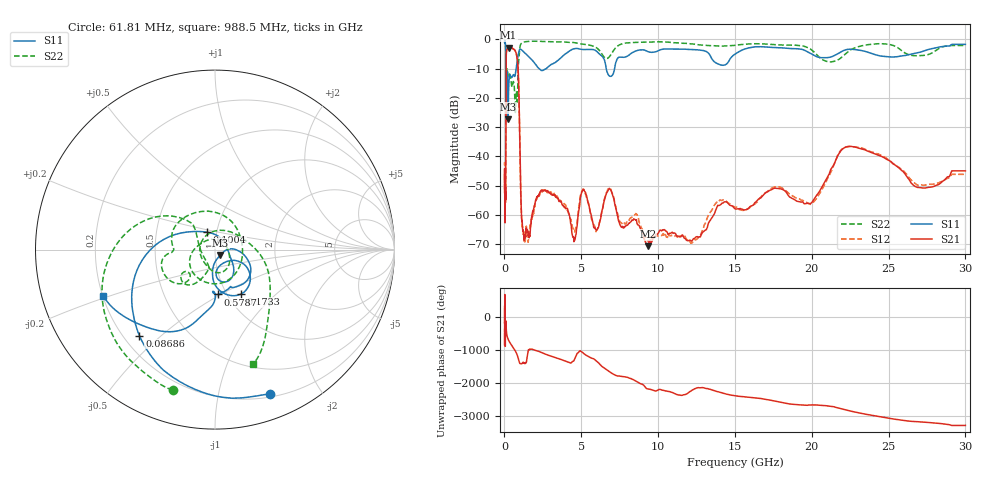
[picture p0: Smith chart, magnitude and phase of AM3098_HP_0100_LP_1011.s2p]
! Date/Time: Thu, Feb 28, 2019 8:35 AM
! Network Analyzer: Agilent Technologies E8364B Rev: A.07.50.67
! Sweep from 0.010 to 30.000 GHz, 1601 Points, Sweep Type: LOG
! Power Supply: 5.022 V, 0.002 A
# Hz S DB R 50
!freq MagS11 AngS11 MagS21 AngS21 MagS12 AngS12 MagS22 AngS22
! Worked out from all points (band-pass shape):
!   1601 points, 10 MHz to 30 GHz, reference 50 ohm
!   highest |S21| = -2.82 dB at 270.5 MHz (marker M1); lowest = -70.7 dB at 9.349 GHz (marker M2)
!   |S21| within 3 dB of the highest: 112.1 MHz to 807.5 MHz (695.4 MHz wide, 151 % of centre)
!   lowest |S11| = -27.4 dB at 235.1 MHz (marker M3), VSWR 1.09, Z = 53.1 - j3.2 ohm
!   |S11| at or under -10 dB: 95.98 MHz to 756.7 MHz (660.7 MHz wide, 155 % of centre); 2.27 GHz to 2.709 GHz (438.8 MHz wide, 17.6 % of centre); 6.627 GHz to 7.167 GHz (539.8 MHz wide, 7.83 % of centre)
!   |S22| runs from -24.9 to -0.6 dB; largest |S21 - S12| = 0.013
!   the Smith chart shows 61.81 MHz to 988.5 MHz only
!   S11 on the Smith chart (normalised r, x): 61.81 MHz: 0.23, -1.43; 86.86 MHz: 0.26, -0.43; 100.4 MHz: 0.90, +0.18; 173.3 MHz: 1.16, -0.63; 578.7 MHz: 0.91, -0.49; 988.5 MHz: 0.20, -0.19
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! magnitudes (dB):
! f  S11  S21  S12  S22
! 10 MHz  -0.3  -46.1  -43.0  -0.6
! 38.04 MHz  -0.5  -57.3  -58.7  -1.0
! 61.81 MHz  -1.3  -51.4  -52.4  -1.7
! 77.03 MHz  -2.2  -53.7  -51.5  -2.6
! 86.86 MHz  -3.9  -36.3  -36.0  -4.3
! 100.4 MHz  -19.4  -11.1  -11.1  -21.9
! 144.7 MHz  -16.7  -3.6  -3.6  -13.6
! 173.3 MHz  -10.8  -3.4  -3.4  -10.1
! 235.1 MHz  -27.4  -2.9  -2.9  -12.4
! 270.5 MHz  -17.0  -2.8  -2.8  -12.7
! 550.5 MHz  -12.2  -3.2  -3.2  -14.6
! 578.7 MHz  -12.0  -3.3  -3.2  -14.4
! 859.3 MHz  -6.3  -8.1  -8.1  -17.6
! 988.5 MHz  -3.4  -32.7  -32.7  -3.4
! 1.093 GHz  -3.5  -57.4  -58.6  -1.4
! 1.244 GHz  -4.2  -66.7  -66.4  -0.9
! 2.084 GHz  -8.9  -54.1  -54.4  -0.6
! 7.926 GHz  -5.9  -63.5  -62.9  -1.2
! 9.349 GHz  -4.2  -70.7  -68.7  -0.9
! 19.8 GHz  -4.4  -56.1  -56.0  -3.0
! 22.67 GHz  -3.4  -36.7  -36.7  -3.2
! 30 GHz  -1.7  -44.9  -46.1  -2.1
